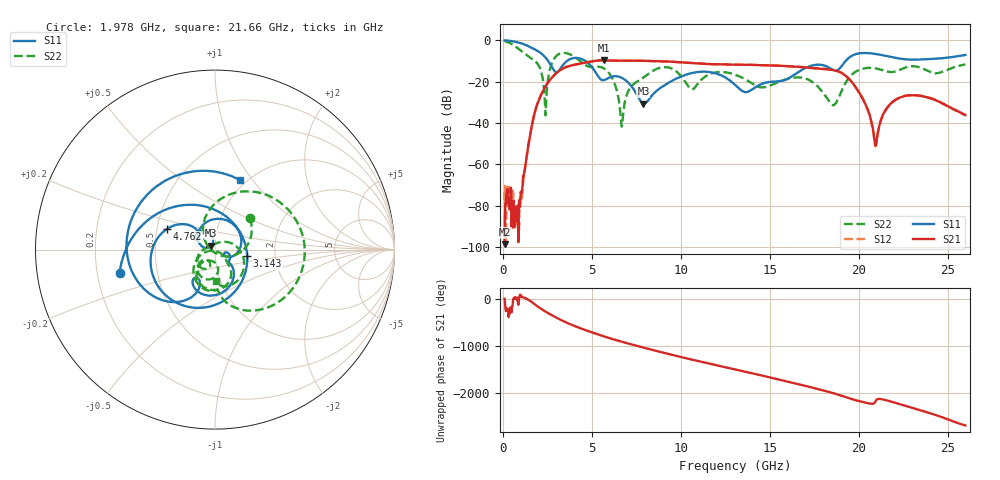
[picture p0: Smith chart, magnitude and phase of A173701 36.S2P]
!  2-Port S-parameters saved by WinCal
! VAR MeasName=S-Parameters (CALIBRATED_DATA) read from VNA (N5245A)
! VAR MeasDate=2017-6-7 10:30:49
! VAR NAME=A173701 36
! VAR FILENAME=A173701 36.S2P
! VAR DATE=2017-6-7 10:30:49
! VAR PHYS_PORTS=1,2
# Hz S DB R 50
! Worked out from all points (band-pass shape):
!   801 points, 100 MHz to 26 GHz, reference 50 ohm
!   highest |S21| = -9.64 dB at 5.668 GHz (marker M1); lowest = -98.7 dB at 100 MHz (marker M2)
!   |S21| within 3 dB of the highest: 3.643 GHz to 16.29 GHz (12.65 GHz wide, 127 % of centre)
!   lowest |S11| = -30.6 dB at 7.902 GHz (marker M3), VSWR 1.06, Z = 48 + j2.06 ohm
!   |S11| at or under -10 dB: 2.551 GHz to 3.597 GHz (1.046 GHz wide, 34 % of centre); 4.65 GHz to 19.26 GHz (14.61 GHz wide, 122 % of centre)
!   |S22| runs from -41.8 to -0.2 dB; largest |S21 - S12| = 0.0048
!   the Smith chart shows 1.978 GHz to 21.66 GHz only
!   S11 on the Smith chart (normalised r, x): 1.978 GHz: 0.30, -0.11; 3.143 GHz: 1.43, -0.11; 4.762 GHz: 0.57, +0.14; 21.66 GHz: 0.93, +0.87
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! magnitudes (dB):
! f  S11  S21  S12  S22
! 100 MHz  0.0  -98.7  -77.1  -0.2
! 941.8 MHz  -1.2  -79.9  -77.2  -4.5
! 1.978 GHz  -5.2  -29.9  -29.9  -11.6
! 2.399 GHz  -8.3  -22.3  -22.3  -36.3
! 3.143 GHz  -14.7  -14.9  -14.9  -6.6
! 4.438 GHz  -9.0  -11.1  -11.1  -10.6
! 4.762 GHz  -10.7  -10.5  -10.5  -12.5
! 5.668 GHz  -19.3  -9.6  -9.7  -13.5
! 6.705 GHz  -18.2  -9.8  -9.8  -41.5
! 7.093 GHz  -20.8  -9.8  -9.8  -23.9
! 7.902 GHz  -30.6  -9.9  -9.9  -18.0
! 8.744 GHz  -23.7  -10.1  -10.1  -13.5
! 10.62 GHz  -15.8  -10.9  -11.0  -23.7
! 13.05 GHz  -21.4  -11.7  -11.7  -16.6
! 17.39 GHz  -12.1  -13.4  -13.3  -20.1
! 18.59 GHz  -14.4  -14.4  -14.3  -31.4
! 19.52 GHz  -7.9  -19.3  -19.2  -17.4
! 20.95 GHz  -6.6  -51.1  -51.1  -13.5
! 21.66 GHz  -7.7  -31.9  -32.1  -15.2
! 21.69 GHz  -7.8  -31.6  -31.7  -15.2
! 23.41 GHz  -9.3  -26.8  -26.7  -13.0
! 26 GHz  -7.0  -36.2  -36.1  -11.7
